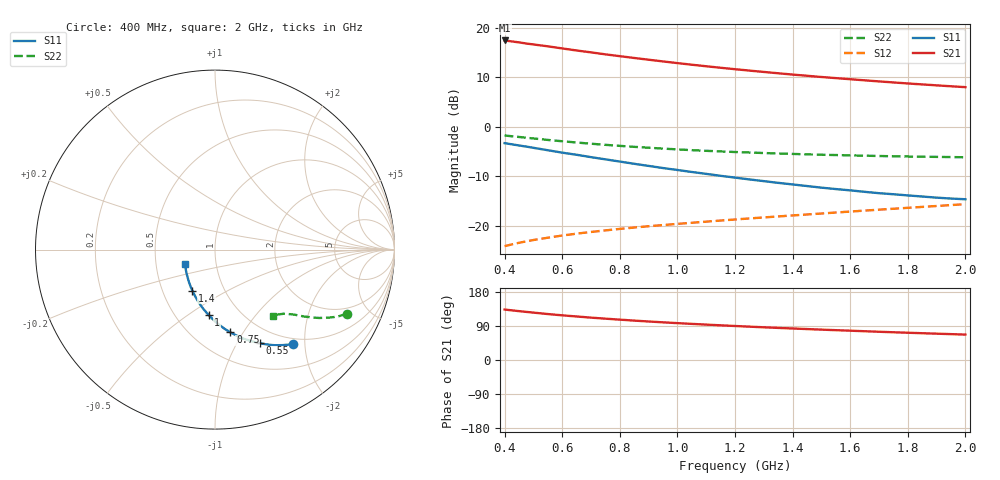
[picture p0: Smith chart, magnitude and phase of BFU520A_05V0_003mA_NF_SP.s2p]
! Filename:  P:\Prog\Test\Noise\ATS_data\Testdata_Net\06 Compressed Noise after Statistics\BFU520A_APG2013_30_A05_05p0V_003mA_NF_CM01_D.sf
! Date/Time: Wed 24/Apr/2013 20:06:17
! BFU520A_APG2013_30_A05_05p0V_1to20mA_NF_CM01_Bias3_R.sf
! Noise Parameter Data File
! BFU520A_APG2013_30_A05_05p0V_1to20mA_NF_CM01
! Date/time: Thu Apr 11 01:07:08 2013
! VAR V_out= 5.001000
! VAR I_out= 3.000000
! VAR V_in= 0.818800
! VAR I_in= 0.032510
! Device data file deembeded for feedlines and parallel
! Original file: \06 Compressed Noise after Statistics\BFU520A_APG2013_30_A05_05p0V_003mA_NF_CM01_R.sf
! Feed-files: PR017V01_150413_Feed1.s2p, PR017V01_150413_Feed2.s2p
! Parallel-file: PR017V01_150413_Par.s2p
# MHz S MA R 50
!  Freq-MHz  S11-mag  S11-arg  S21-mag  S21-arg  S12-mag  S12-arg  S22-mag  S22-arg
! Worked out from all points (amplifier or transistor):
!   37 points, 400 MHz to 2 GHz, reference 50 ohm
!   highest |S21| = 17.5 dB at 400 MHz (marker M1)
!   |S21| within 3 dB of that: start of sweep to 775.9 MHz
!   unconditionally stable (mu >= 1): 1.863 GHz to end of sweep
!   at 500 MHz: K = 0.46, MSG = 19.8 dB, |S12| = -22.9 dB
!   at 1.1 GHz: K = 0.82, MSG = 15.7 dB, |S12| = -19.2 dB
!   at 2 GHz: K = 1.01, MAG = 11.2 dB, |S12| = -15.6 dB
!   lowest NFmin = 0.59 dB at 440 MHz
!   S11 on the Smith chart (normalised r, x): 400 MHz: 0.90, -1.77; 550 MHz: 0.80, -1.25; 750 MHz: 0.74, -0.88; 1 GHz: 0.72, -0.60; 1.4 GHz: 0.71, -0.35; 2 GHz: 0.71, -0.12
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400  0.6832 -50.4  7.467 133.2  0.06206 64.6  0.8165 -26.0
420  0.6686 -52.4  7.337 131.4  0.06414 63.8  0.8052 -26.8
460  0.6405 -56.2  7.067 128.2  0.06807 62.6  0.784 -28.2
500  0.613 -60.0  6.805 125.0  0.07163 61.5  0.7626 -29.5
550  0.5794 -64.4  6.512 121.3  0.07562 60.3  0.7366 -31.0
600  0.5478 -68.6  6.202 117.9  0.07948 59.4  0.7142 -32.2
650  0.5213 -72.2  5.911 114.8  0.08308 58.6  0.6937 -33.3
700  0.4933 -76.0  5.659 111.8  0.08641 58.1  0.6745 -34.2
750  0.4687 -79.5  5.403 109.1  0.08963 57.6  0.6571 -35.1
800  0.4451 -83.0  5.179 106.5  0.09276 57.4  0.6414 -35.8
850  0.4224 -86.3  4.966 104.0  0.09579 57.1  0.627 -36.6
900  0.4024 -89.6  4.769 101.6  0.09875 56.9  0.6144 -37.2
950  0.3827 -92.7  4.581 99.4  0.1015 56.9  0.6017 -37.8
1000  0.3659 -95.6  4.407 97.3  0.1043 56.9  0.5911 -38.4
1100  0.3342 -101.7  4.095 93.4  0.1098 57.1  0.5715 -39.4
1200  0.3064 -107.4  3.824 89.7  0.1155 57.4  0.5559 -40.4
1300  0.2822 -113.1  3.588 86.3  0.1211 57.7  0.543 -41.4
1400  0.2613 -118.9  3.374 83.2  0.1269 58.1  0.5318 -42.4
1500  0.2425 -124.8  3.19 80.2  0.1327 58.6  0.5216 -43.3
1650  0.22 -133.4  2.952 75.9  0.1421 59.2  0.5106 -44.9
1750  0.2079 -139.6  2.808 73.2  0.1483 59.6  0.5037 -45.9
2000  0.1851 -154.6  2.518 67.0  0.165 60.5  0.492 -48.8
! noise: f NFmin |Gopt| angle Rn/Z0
400  0.6121  0.3569  14.97  0.1671
460  0.6127  0.3423  21.96  0.1556
600  0.7  0.3517  21.52  0.1779
800  0.6505  0.318  37.94  0.143
1000  0.7013  0.3078  50.49  0.1308
1200  0.7375  0.3033  59.95  0.131
1400  0.7792  0.2703  74.36  0.1159
1600  0.788  0.2534  84.03  0.1024
1800  0.6966  0.2616  109.3  0.0868
2000  0.821  0.2384  111.4  0.0805
